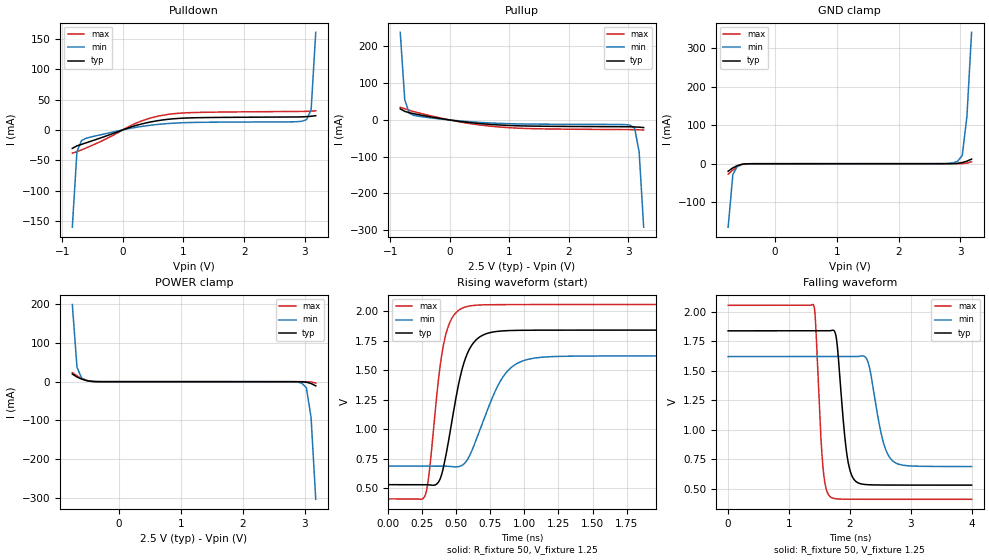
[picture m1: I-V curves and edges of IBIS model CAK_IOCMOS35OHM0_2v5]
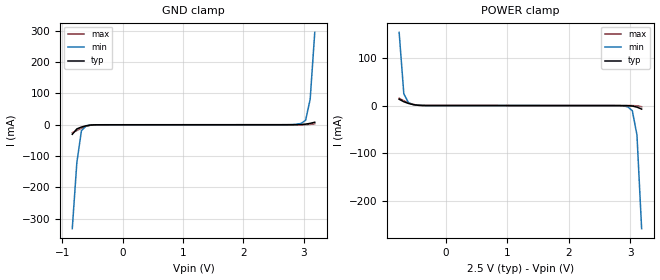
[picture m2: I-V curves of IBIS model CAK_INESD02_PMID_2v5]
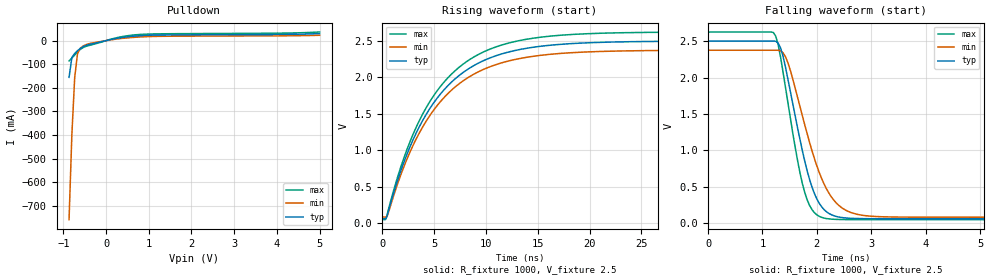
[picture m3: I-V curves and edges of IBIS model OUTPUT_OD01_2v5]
|   This file is an IBIS representation of the   |
|   Integrated Device Technology, Inc.   |
|   IDT8T49N241I   |
|   FEMTOCLOCK NG SINGLE UNIVERSAL FREQUENCY TRANSLATOR   |
[IBIS Ver]   4.1
[File name]   8t49n241i.ibs
[File Rev]   1.0
[Date]   9 Apr 2015
[Source]   Originated at Integrated Device Technology, Inc.
[Notes] This model is a based on preliminary lab data.  Typical conditions
have been correlated to lab data.  Minimum and Maximum conditions have
not been correlated to characterization data.
[Disclaimer]
IDT hereby grants the user of this IBIS model a non-exclusive,
nontransferable license to use this IBIS model under the following terms.
Before using this IBIS model, the user should read this license.
If the user does not accept these terms,  the IBIS model should be
returned to IDT within 30 days.
   The user is granted this license only to use the IBIS model and
is not granted rights to sell, load, rent, lease or license the IBIS
model in whole or in part, or in modified form to anyone other than
user. User may modify the IBIS model to suit its specific
applications but rights to derivative works and such modifications
shall belong to IDT.
   This IBIS model is provided on an "AS IS" basis and IDT makes
absolutely no warranty with respect to the information contained
herein. IDT DISCLAIMS AND CUSTOMER WAIVES ALL WARRANTIES, EXPRESS
OR IMPLIED, INCLUDING WARRANTIES OF MERCHANTABILITY OR FITNESS FOR
A PARTICULAR PURPOSE. The entire risk as to quality and performance
is with the Customer. ACCORDINGLY, IN NO EVENT SHALL THE COMPANY BE
LIABLE FOR ANY DAMAGES, WHETHER IN CONTRACT OR TORT,INCLUDING ANY
LOST PROFITS OR OTHER INCIDENTAL, CONSEQUENTIAL, EXEMPLARY, OR
PUNITIVE DAMAGES ARISING OUT OF THE USE OR APPLICATION OF THE IBIS
model provided in this package. Further, IDT reserves the right to
make changes without notice to any product herein to improve
reliability, function, or design. IDT does not convey any license
under patent rights or any other intellectual property rights,
including those of third parties.
   IDT is not obligated to provide maintenance or support
for the licensed IBIS model.
[Copyright] Copyright 2015 by Integrated Device Technology, Inc.
[Component]   IDT8T49N241NLGI
[Manufacturer] Integrated Device Technology, Inc.
[Package]
|LD QFN 40
|lead + wire   typ   min   max
R_pkg   7.1539E-02   5.8459E-02   9.5092E-02
L_pkg   1.4325E-09   1.0877E-09   2.0537E-09
C_pkg   5.9801E-14   5.5325E-14   6.5653E-14
[Pin] signal_name  model_name   R_pin   L_pin   C_pin
1   VCCA   POWER   8.5557E-02   1.8029E-09   6.3191E-14
2   VCCA   POWER   7.6183E-02   1.5542E-09   6.2015E-14
3   GPIO[0]   CAK_IOCMOS25OHM0   6.6383E-02   1.2964E-09   5.8526E-14
4   VCCO0   POWER   6.6920E-02   1.3109E-09   5.8763E-14
5   Q0   OCELL_CMOS_PECL_   6.0741E-02   1.1478E-09   5.6176E-14
6   nQ0   OCELL_CMOS_PECL_   5.8459E-02   1.0877E-09   5.5325E-14
7   GIPO[1]   CAK_IOCMOS25OHM0   6.0207E-02   1.1343E-09   5.6120E-14
8   nQ1   OCELL_CMOS_PECL_   6.3964E-02   1.2328E-09   5.7694E-14
9   Q1   OCELL_CMOS_PECL_   7.1615E-02   1.4340E-09   6.0514E-14
10  VCCO1   POWER   8.6096E-02   1.8170E-09   6.3252E-14
11  SDATA   CAK_IOCMOS35OHM0   8.6631E-02   1.8312E-09   6.3484E-14
12  SCLK   CAK_IOCMOS35OHM0   7.5512E-02   1.5366E-09   6.1638E-14
13  VCC   POWER   6.6247E-02   1.2928E-09   5.8380E-14
14  VEE   GND   6.0743E-02   1.1484E-09   5.6429E-14
15  VCC   POWER   5.9668E-02   1.1195E-09   5.5855E-14
16  CLK0   CAK_INESD02_PD   6.3966E-02   1.2326E-09   5.7537E-14
17  nCLKO   CAK_INESD02_PMID   7.3233E-02   1.4771E-09   6.1020E-14
18  CLK1   CAK_INESD02_PD   8.2496E-02   1.7204E-09   6.3925E-14
19  nCLK1   CAK_INESD02_PMID   8.5045E-02   1.7874E-09   6.4649E-14
20  S_A1   CAK_INESD01_PD   9.5092E-02   2.0537E-09   6.5653E-14
21  VCCO2   POWER   8.6362E-02   1.8241E-09   6.3205E-14
22  Q2   OCELL_CMOS_PECL_   7.0946E-02   1.4164E-09   6.0237E-14
23  nQ2   OCELL_CMOS_PECL_   6.8663E-02   1.3564E-09   5.9445E-14
24  GPIO[2]   CAK_IOCMOS25OHM0   6.5040E-02   1.2614E-09   5.8000E-14
25  nQ3   OCELL_CMOS_PECL_   6.0742E-02   1.1479E-09   5.6257E-14
26  Q3   OCELL_CMOS_PECL_   6.1547E-02   1.1691E-09   5.6462E-14
27  VCCO3   POWER   6.4102E-02   1.2369E-09   5.7655E-14
28  GPIO[3]   CAK_IOCMOS25OHM0   6.7053E-02   1.3140E-09   5.8813E-14
29  nINT   OUTPUT_OD01   7.2958E-02   1.4693E-09   6.1096E-14
30  VCCA   POWER   8.6901E-02   1.8381E-09   6.3478E-14
31  nRST   CAK_INESD01_PU   8.9987E-02   1.9196E-09   6.4336E-14
32  VCCA   POWER   8.0749E-02   1.6744E-09   6.3449E-14
33  OSCI   CAK_INESD01   6.9197E-02   1.3705E-09   5.9552E-14
34  OSCO   NC   7.0009E-02   1.3922E-09   6.0035E-14
35  nWP   CAK_INESD01_PU   6.1145E-02   1.1585E-09   5.6415E-14
36  VCCCS   POWER   5.9937E-02   1.1266E-09   5.5909E-14
37  CAP   NC   5.9804E-02   1.1237E-09   5.5979E-14
38  CAP_REF   NC   6.5441E-02   1.2716E-09   5.8175E-14
39  VCCA   POWER   7.3496E-02   1.4835E-09   6.1056E-14
40  S_A0   CAK_INESD01_PD   8.2738E-02   1.7286E-09   6.2354E-14
41  EPAD   GND
[Diff Pin]  inv_pin  vdiff tdelay_typ tdelay_min  tdelay_max
16   17   0.15   NA   NA   NA
18   19   0.15   NA   NA   NA
5   6   NA   0   0   0
9   8   NA   0   0   0
22   23   NA   0   0   0
26   25   NA   0   0   0
[Model Selector] CAK_IOCMOS25OHM0
CAK_IOCMOS25OHM0_2v5  Buffer selection for 2v5
CAK_IOCMOS25OHM0_3v3  Buffer selection for 3v3
[Model Selector] OCELL_CMOS_PECL_
OCELL_LVPECL_2v5  2.5V LVPECL Driver
OCELL_LVPECL_3v3  3.3V LVPECL Driver
OCELL_LVDS_2v5   2.5V LVDS Driver
OCELL_LVDS_3v3   3.3V LVDS Driver
OCELL_LVCMOS_1v8  1.8V LVCMOS Driver
OCELL_LVCMOS_2v5  2.5V LVCMOS Driver
OCELL_LVCMOS_3v3  3.3V LVCMOS Driver
OCELL_HCSL_2v5   2.5V HCSL Driver
OCELL_HCSL_3v3   3.3V HCSL Driver
[Model Selector] CAK_IOCMOS35OHM0
CAK_IOCMOS35OHM0_2v5  Buffer selection for 2v5
CAK_IOCMOS35OHM0_3v3  Buffer selection for 3v3
[Model Selector] CAK_INESD02_PD
CAK_INESD02_PD_2v5  Buffer selection for 2v5
CAK_INESD02_PD_3v3  Buffer selection for 3v3
[Model Selector] CAK_INESD02_PMID
CAK_INESD02_PMID_2v5  Buffer selection for 2v5
CAK_INESD02_PMID_3v3  Buffer selection for 3v3
[Model Selector] CAK_INESD01_PD
CAK_INESD01_PD_2v5  Buffer selection for 2v5
CAK_INESD01_PD_3v3  Buffer selection for 3v3
[Model Selector] OUTPUT_OD01
OUTPUT_OD01_2v5  Buffer selection for 2v5
OUTPUT_OD01_3v3  Buffer selection for 3v3
[Model Selector] CAK_INESD01_PU
CAK_INESD01_PU_2v5  Buffer selection for 2v5
CAK_INESD01_PU_3v3  Buffer selection for 3v3
[Model Selector] CAK_INESD01
CAK_INESD01_2v5  Buffer selection for 2v5
CAK_INESD01_3v3  Buffer selection for 3v3
| Models and submodels in the file (25): CAK_IOCMOS25OHM0_2v5 (Input), CAK_IOCMOS35OHM0_2v5 (I/O), CAK_INESD02_PD_2v5 (Input), CAK_INESD02_PMID_2v5 (Input), CAK_INESD01_PD_2v5 (Input), OUTPUT_OD01_2v5 (Open_drain), CAK_INESD01_PU_2v5 (Input), CAK_INESD01_2v5 (Input), CAK_IOCMOS25OHM0_3v3 (Input), OCELL_LVPECL_2v5 (Output_ECL), OCELL_LVPECL_3v3 (Output_ECL), OCELL_LVDS_2v5 (Output), OCELL_LVDS_3v3 (Output), OCELL_LVCMOS_1v8 (Output), OCELL_LVCMOS_2v5 (Output), OCELL_LVCMOS_3v3 (Output), OCELL_HCSL_2v5 (Open_source), OCELL_HCSL_3v3 (Open_source), CAK_IOCMOS35OHM0_3v3 (Output), CAK_INESD02_PD_3v3 (Input), CAK_INESD02_PMID_3v3 (Input), CAK_INESD01_PD_3v3 (Input), OUTPUT_OD01_3v3 (Open_drain), CAK_INESD01_PU_3v3 (Input), CAK_INESD01_3v3 (Input)
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| 3.18182e+00   -1.19855e-02   -3.78182e-01   -3.86041e-03
| 3.25758e+00   -2.18155e-02   -9.33967e-01   -1.12351e-02
| 3.33333e+00   -5.03193e-02   -1.56445e+00   -2.21741e-02
| 3.40909e+00   -2.87346e-01   -2.19530e+00   -3.46613e-02
| 3.48485e+00   -9.49059e-01   -2.82642e+00   -4.62600e-02
| 3.56061e+00   -1.79228e+00   -3.45775e+00   -9.04319e-02
| 3.63636e+00   -2.63582e+00   -4.08929e+00   -5.29971e-01
| 3.71212e+00   -3.47965e+00   -4.72100e+00   -1.58901e+00
| 3.78788e+00   -4.32375e+00   -5.35288e+00   -2.66834e+00
| 3.86364e+00   -5.16810e+00   -5.98493e+00   -3.74797e+00
| 3.93939e+00   -6.01268e+00   -6.61714e+00   -4.82785e+00
| 4.01515e+00   -6.85746e+00   -7.24950e+00   -5.90795e+00
| 4.09091e+00   -7.70243e+00   -7.88200e+00   -6.98824e+00
| 4.16667e+00   -8.54757e+00   -8.51465e+00   -8.06870e+00
| 4.24242e+00   -9.39286e+00   -9.14742e+00   -9.14928e+00
| 4.31818e+00   -1.02383e+01   -9.78033e+00   -1.02300e+01
| 4.39394e+00   -1.10838e+01   -1.04133e+01   -1.13108e+01
| 4.46970e+00   -1.19295e+01   -1.10465e+01   -1.23917e+01
| 4.54545e+00   -1.27752e+01   -1.16797e+01   -1.34727e+01
| 4.62121e+00   -1.36211e+01   -1.23131e+01   -1.45537e+01
| 4.69697e+00   -1.44670e+01   -1.29465e+01   -1.56349e+01
| 4.77273e+00   -1.53129e+01   -1.35800e+01   -1.67160e+01
| 4.84848e+00   -1.61590e+01   -1.42136e+01   -1.77972e+01
| 4.92424e+00   -1.70051e+01   -1.48473e+01   -1.88785e+01
| 5.00000e+00   -1.78512e+01   -1.54810e+01   -1.99597e+01
[Model] CAK_IOCMOS35OHM0_2v5
Model_type   I/O
Polarity   Non-Inverting
|   typ   min   max
C_comp   2pF   1.5pF   2.5pF
|Input
Vinl = 0.7V
Vinh = 1.7V
|Output
Vmeas = 1.25V
Rref = 50
Cref = 0
Vref = 1.25V
|   typ   min   max
[Voltage range]   2.5V   2.375V   2.625V
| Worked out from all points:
|   slope of the pulldown table from 0 to 0.375 V, typ, clamps not added: 33.2 ohm
|   slope of the pullup table from 0 to 0.375 V, typ, clamps not added: 48.8 ohm
|   GND clamp passes 1 mA (typ) near -0.50 V on its own axis
|   POWER clamp passes 1 mA (typ) near -0.46 V on its own axis
|   rising waveform, R_fixture 50, V_fixture 1.25: 20-80 % time 134ps typ, 204ps min, 96.8ps max; typ from 0.531 V to 1.84 V
|   falling waveform, R_fixture 50, V_fixture 1.25: 20-80 % time 134ps typ, 204ps min, 95ps max; typ from 1.84 V to 0.531 V
[GND_clamp]
|Voltage   I (typ)   I (min)   I (max)
|Note, modeling breaks down at 250mA and above.  This is well beyond the functional   |
|operating range of the device.  Should this scenario occur, catastrophic failure and   |
|possible damage to the device and/or board is of higher concern than the I-V curve   |
|behavior.  The IBIS checker will flag currents in excess of 10A with warnings.  Lines   |
|with currents in excess of 0.35 A have been commented out.  The points still remain|
|available to the user if the user desires to use them.   |
|-2.42424e+00   -5.99088e+00   -4.88415e+00   -7.24880e+00
|-2.34848e+00   -5.70272e+00   -4.66840e+00   -6.88094e+00
|-2.27273e+00   -5.41462e+00   -4.45272e+00   -6.51310e+00
|-2.19697e+00   -5.12656e+00   -4.23712e+00   -6.14529e+00
|-2.12121e+00   -4.83856e+00   -4.02161e+00   -5.77750e+00
|-2.04545e+00   -4.55064e+00   -3.80620e+00   -5.40975e+00
|-1.96970e+00   -4.26278e+00   -3.59088e+00   -5.04205e+00
|-1.89394e+00   -3.97502e+00   -3.37567e+00   -4.67441e+00
|-1.81818e+00   -3.68735e+00   -3.16057e+00   -4.30683e+00
|-1.74242e+00   -3.39979e+00   -2.94558e+00   -3.93934e+00
|-1.66667e+00   -3.11235e+00   -2.73072e+00   -3.57193e+00
|-1.59091e+00   -2.82505e+00   -2.51599e+00   -3.20462e+00
|-1.51515e+00   -2.53790e+00   -2.30139e+00   -2.83743e+00
|-1.43939e+00   -2.25092e+00   -2.08694e+00   -2.47036e+00
|-1.36364e+00   -1.96413e+00   -1.87263e+00   -2.10344e+00
|-1.28788e+00   -1.67754e+00   -1.65847e+00   -1.73670e+00
|-1.21212e+00   -1.39118e+00   -1.44447e+00   -1.37017e+00
|-1.13636e+00   -1.10506e+00   -1.23064e+00   -1.00389e+00
|-1.06061e+00   -8.19198e-01   -1.01701e+00   -6.37879e-01
|-9.84848e-01   -5.33627e-01   -8.03591e-01   -2.72184e-01
|-9.09091e-01   -2.48371e-01   -5.90465e-01   -5.58283e-02
|-8.33333e-01   -4.53732e-02   -3.77762e-01   -3.79192e-02
-757.6mV  -19.7mA    -165.1mA   -27.4mA
-681.8mV  -10.83mA   -28.37mA   -16.29mA
-606.1mV  -4.786mA   -6.047mA   -7.399mA
-530.3mV  -1.407mA   -1.506mA   -2.105mA
-378.8mV  -80.75uA   -97.08uA   -91.06uA
2.727V    4.903uA    107uA      2.354uA
2.879V    114.3uA    2.196mA    6.393uA
2.955V    801.8uA    6.121mA    22.36uA
3.03V     2.877mA    21.15mA    238.2uA
3.106V    6.558mA    121.9mA    1.646mA
3.182V    11.89mA    341.6mA    5.038mA
| 3.25758e+00   1.96472e-02   5.60110e-01   1.04123e-02
| 3.33333e+00   4.87507e-02   7.78570e-01   1.76749e-02
| 3.40909e+00   2.77107e-01   9.97201e-01   2.56783e-02
| 3.48485e+00   5.68788e-01   1.21604e+00   3.28468e-02
| 3.56061e+00   8.60732e-01   1.43508e+00   7.83400e-02
| 3.63636e+00   1.15296e+00   1.65434e+00   4.20975e-01
| 3.71212e+00   1.44548e+00   1.87382e+00   7.94432e-01
| 3.78788e+00   1.73828e+00   2.09351e+00   1.16825e+00
| 3.86364e+00   2.03137e+00   2.31341e+00   1.54243e+00
| 3.93939e+00   2.32473e+00   2.53352e+00   1.91695e+00
| 4.01515e+00   2.61836e+00   2.75385e+00   2.29181e+00
| 4.09091e+00   2.91225e+00   2.97438e+00   2.66701e+00
| 4.16667e+00   3.20641e+00   3.19513e+00   3.04252e+00
| 4.24242e+00   3.50082e+00   3.41608e+00   3.41834e+00
| 4.31818e+00   3.79548e+00   3.63725e+00   3.79446e+00
| 4.39394e+00   4.09039e+00   3.85863e+00   4.17087e+00
| 4.46970e+00   4.38554e+00   4.08023e+00   4.54756e+00
| 4.54545e+00   4.68094e+00   4.30204e+00   4.92452e+00
| 4.62121e+00   4.97658e+00   4.52407e+00   5.30175e+00
| 4.69697e+00   5.27245e+00   4.74633e+00   5.67924e+00
| 4.77273e+00   5.56857e+00   4.96881e+00   6.05699e+00
| 4.84848e+00   5.86492e+00   5.19152e+00   6.43499e+00
| 4.92424e+00   6.16151e+00   5.41446e+00   6.81323e+00
| 5.00000e+00   6.45834e+00   5.63765e+00   7.19172e+00
[Power_clamp]
|Voltage   I (typ)   I (min)   I (max)
|Note, modeling breaks down at 250mA and above.  This is well beyond the functional   |
|operating range of the device.  Should this scenario occur, catastrophic failure and   |
|possible damage to the device and/or board is of higher concern than the I-V curve   |
|behavior.  The IBIS checker will flag currents in excess of 10A with warnings.  Lines   |
|with currents in excess of 0.35 A have been commented out.  The points still remain|
|available to the user if the user desires to use them.   |
|-2.42424e+00   6.16151e+00   5.04673e+00   7.43787e+00
|-2.34848e+00   5.86492e+00   4.82417e+00   7.05922e+00
|-2.27273e+00   5.56857e+00   4.60184e+00   6.68082e+00
|-2.19697e+00   5.27245e+00   4.37973e+00   6.30266e+00
|-2.12121e+00   4.97658e+00   4.15784e+00   5.92475e+00
|-2.04545e+00   4.68094e+00   3.93617e+00   5.54709e+00
|-1.96970e+00   4.38554e+00   3.71471e+00   5.16969e+00
|-1.89394e+00   4.09039e+00   3.49347e+00   4.79255e+00
|-1.81818e+00   3.79548e+00   3.27244e+00   4.41568e+00
|-1.74242e+00   3.50082e+00   3.05162e+00   4.03909e+00
|-1.66667e+00   3.20641e+00   2.83101e+00   3.66278e+00
|-1.59091e+00   2.91225e+00   2.61061e+00   3.28677e+00
|-1.51515e+00   2.61836e+00   2.39042e+00   2.91105e+00
|-1.43939e+00   2.32473e+00   2.17045e+00   2.53565e+00
|-1.36364e+00   2.03137e+00   1.95069e+00   2.16057e+00
|-1.28788e+00   1.73828e+00   1.73114e+00   1.78583e+00
|-1.21212e+00   1.44548e+00   1.51180e+00   1.41142e+00
|-1.13636e+00   1.15296e+00   1.29268e+00   1.03737e+00
|-1.06061e+00   8.60732e-01   1.07377e+00   6.63681e-01
|-9.84848e-01   5.68788e-01   8.55069e-01   2.90350e-01
|-9.09091e-01   2.77107e-01   6.36557e-01   4.68087e-02
|-8.33333e-01   4.87507e-02   4.18123e-01   3.00765e-02
-757.6mV  19.65mA    199mA      23mA
-681.8mV  11.89mA    37.01mA    14.94mA
-606.1mV  6.558mA    8.981mA    8.308mA
-530.3mV  2.877mA    3.169mA    3.622mA
-303mV    14.46uA    30.61uA    12.18uA
2.727V    -54.42uA   -72.56uA   -62.76uA
2.879V    -80.75uA   -908.8uA   -66.34uA
2.955V    -281.2uA   -3.717mA   -70.88uA
3.03V     -1.407mA   -15.93mA   -127.8uA
3.106V    -4.786mA   -92.25mA   -684.1uA
3.182V    -10.83mA   -303.4mA   -3.499mA
| 3.25758e+00   -1.96989e-02   -5.15962e-01   -1.01554e-02
| 3.33333e+00   -4.53732e-02   -7.28958e-01   -2.00234e-02
| 3.40909e+00   -2.48371e-01   -9.42283e-01   -3.12866e-02
| 3.48485e+00   -5.33627e-01   -1.15585e+00   -4.17513e-02
| 3.56061e+00   -8.19198e-01   -1.36961e+00   -8.15325e-02
| 3.63636e+00   -1.10506e+00   -1.58355e+00   -4.00139e-01
| 3.71212e+00   -1.39118e+00   -1.79765e+00   -7.65947e-01
| 3.78788e+00   -1.67754e+00   -2.01191e+00   -1.13206e+00
| 3.86364e+00   -1.96413e+00   -2.22632e+00   -1.49843e+00
| 3.93939e+00   -2.25092e+00   -2.44086e+00   -1.86504e+00
| 4.01515e+00   -2.53790e+00   -2.65555e+00   -2.23184e+00
| 4.09091e+00   -2.82505e+00   -2.87037e+00   -2.59881e+00
| 4.16667e+00   -3.11235e+00   -3.08531e+00   -2.96593e+00
| 4.24242e+00   -3.39979e+00   -3.30037e+00   -3.33317e+00
| 4.31818e+00   -3.68735e+00   -3.51555e+00   -3.70052e+00
| 4.39394e+00   -3.97502e+00   -3.73083e+00   -4.06795e+00
| 4.46970e+00   -4.26278e+00   -3.94621e+00   -4.43548e+00
| 4.54545e+00   -4.55064e+00   -4.16168e+00   -4.80307e+00
| 4.62121e+00   -4.83856e+00   -4.37725e+00   -5.17074e+00
| 4.69697e+00   -5.12656e+00   -4.59290e+00   -5.53846e+00
| 4.77273e+00   -5.41462e+00   -4.80863e+00   -5.90622e+00
| 4.84848e+00   -5.70272e+00   -5.02443e+00   -6.27402e+00
| 4.92424e+00   -5.99088e+00   -5.24031e+00   -6.64184e+00
| 5.00000e+00   -6.27908e+00   -5.45625e+00   -7.00969e+00
[Pulldown]
|Voltage   I (typ)   I (min)   I (max)
|Note, modeling breaks down at 250mA and above.  This is well beyond the functional   |
|operating range of the device.  Should this scenario occur, catastrophic failure and   |
|possible damage to the device and/or board is of higher concern than the I-V curve   |
|behavior.  The IBIS checker will flag currents in excess of 10A with warnings.  Lines   |
|with currents in excess of 0.35 A have been commented out.  The points still remain|
|available to the user if the user desires to use them.   |
|-2.424240e+00   -5.620920e+00   -4.561270e+00   -6.831600e+00
|-2.348480e+00   -5.341380e+00   -4.351820e+00   -6.474360e+00
|-2.272730e+00   -5.061780e+00   -4.142370e+00   -6.117000e+00
|-2.196970e+00   -4.782250e+00   -3.932930e+00   -5.759610e+00
|-2.121210e+00   -4.502700e+00   -3.723470e+00   -5.402300e+00
|-2.045450e+00   -4.223130e+00   -3.514010e+00   -5.044950e+00
|-1.969700e+00   -3.943570e+00   -3.304540e+00   -4.687600e+00
|-1.893940e+00   -3.663980e+00   -3.095070e+00   -4.330220e+00
|-1.818180e+00   -3.384390e+00   -2.885580e+00   -3.972840e+00
|-1.742420e+00   -3.104780e+00   -2.676080e+00   -3.615430e+00
|-1.666670e+00   -2.825150e+00   -2.466570e+00   -3.258010e+00
|-1.590910e+00   -2.545490e+00   -2.257030e+00   -2.900560e+00
|-1.515150e+00   -2.265810e+00   -2.047480e+00   -2.543070e+00
|-1.439390e+00   -1.986090e+00   -1.837900e+00   -2.185550e+00
|-1.363640e+00   -1.706320e+00   -1.628300e+00   -1.827980e+00
|-1.287880e+00   -1.426520e+00   -1.418670e+00   -1.470360e+00
|-1.212120e+00   -1.146650e+00   -1.209020e+00   -1.112660e+00
|-1.136360e+00   -8.667200e-01   -9.993300e-01   -7.548700e-01
|-1.060610e+00   -5.867220e-01   -7.896000e-01   -3.969910e-01
|-9.848480e-01   -3.066460e-01   -5.798390e-01   -7.806800e-02
|-9.090910e-01   -6.551900e-02   -3.700490e-01   -4.152980e-02
-833.3mV  -30.4mA    -160.2mA   -38.37mA
-757.6mV  -26.34mA   -35.84mA   -35.89mA
-681.8mV  -23.84mA   -17.61mA   -32.95mA
-606.1mV  -21.34mA   -13.8mA    -29.8mA
227.3mV   7.551mA    4.361mA    11.42mA
454.5mV   12.99mA    7.63mA     19.37mA
681.8mV   16.67mA    9.951mA    24.52mA
1.212V    20.01mA    12.36mA    28.66mA
2.803V    21.22mA    13.27mA    30.3mA
3.03V     21.8mA     16.76mA    30.5mA
3.106V    22.45mA    33.64mA    30.79mA
3.182V    23.38mA    160.7mA    31.41mA
|3.257580e+00   2.470960e-02   3.762400e-01   3.236290e-02
|3.333330e+00   2.959920e-02   5.918100e-01   3.363400e-02
|3.409090e+00   1.001510e-01   8.074090e-01   3.503170e-02
|3.484850e+00   3.838970e-01   1.023030e+00   3.629400e-02
|3.560610e+00   6.718180e-01   1.238710e+00   4.394800e-02
|3.636360e+00   9.597900e-01   1.454410e+00   2.364620e-01
|3.712120e+00   1.247810e+00   1.670150e+00   6.046980e-01
|3.787880e+00   1.535890e+00   1.885920e+00   9.730100e-01
|3.863640e+00   1.824010e+00   2.101740e+00   1.341380e+00
|3.939390e+00   2.112190e+00   2.317600e+00   1.709840e+00
|4.015150e+00   2.400420e+00   2.533480e+00   2.078370e+00
|4.090910e+00   2.688710e+00   2.749420e+00   2.446960e+00
|4.166670e+00   2.977050e+00   2.965390e+00   2.815630e+00
|4.242420e+00   3.265440e+00   3.181400e+00   3.184380e+00
|4.318180e+00   3.553900e+00   3.397450e+00   3.553210e+00
|4.393940e+00   3.842420e+00   3.613550e+00   3.922130e+00
|4.469700e+00   4.131000e+00   3.829690e+00   4.291130e+00
|4.545450e+00   4.419630e+00   4.045870e+00   4.660220e+00
|4.621210e+00   4.708340e+00   4.262110e+00   5.029450e+00
|4.696970e+00   4.997150e+00   4.478390e+00   5.398660e+00
|4.772730e+00   5.285930e+00   4.694720e+00   5.768110e+00
|4.848480e+00   5.574880e+00   4.911080e+00   6.137610e+00
|4.924240e+00   5.863890e+00   5.127540e+00   6.507170e+00
|5.000000e+00   6.153060e+00   5.344050e+00   6.876880e+00
[Pullup]
|Voltage   I (typ)   I (min)   I (max)
|Note, modeling breaks down at 250mA and above.  This is well beyond the functional   |
|operating range of the device.  Should this scenario occur, catastrophic failure and   |
|possible damage to the device and/or board is of higher concern than the I-V curve   |
|behavior.  The IBIS checker will flag currents in excess of 10A with warnings.  Lines   |
|with currents in excess of 0.35 A have been commented out.  The points still remain|
|available to the user if the user desires to use them.   |
|-2.424240e+00   5.884990e+00   4.790360e+00   7.136830e+00
|-2.348480e+00   5.595580e+00   4.573450e+00   6.766980e+00
|-2.272730e+00   5.306130e+00   4.356560e+00   6.397080e+00
|-2.196970e+00   5.016750e+00   4.139690e+00   6.027240e+00
|-2.121210e+00   4.727390e+00   3.922850e+00   5.657350e+00
|-2.045450e+00   4.438030e+00   3.706020e+00   5.287510e+00
|-1.969700e+00   4.148680e+00   3.489220e+00   4.917710e+00
|-1.893940e+00   3.859340e+00   3.272430e+00   4.547940e+00
|-1.818180e+00   3.570020e+00   3.055660e+00   4.178140e+00
|-1.742420e+00   3.280710e+00   2.838900e+00   3.808350e+00
|-1.666670e+00   2.991410e+00   2.622170e+00   3.438570e+00
|-1.590910e+00   2.702130e+00   2.405450e+00   3.068780e+00
|-1.515150e+00   2.412850e+00   2.188750e+00   2.699010e+00
|-1.439390e+00   2.123580e+00   1.972050e+00   2.329220e+00
|-1.363640e+00   1.834310e+00   1.755360e+00   1.959430e+00
|-1.287880e+00   1.545050e+00   1.538690e+00   1.589620e+00
|-1.212120e+00   1.255770e+00   1.322030e+00   1.219810e+00
|-1.136360e+00   9.665000e-01   1.105370e+00   8.499700e-01
|-1.060610e+00   6.772080e-01   8.887100e-01   4.801090e-01
|-9.848480e-01   3.878980e-01   6.720410e-01   1.143440e-01
|-9.090910e-01   1.026590e-01   4.553330e-01   3.942970e-02
-833.3mV  30.43mA    238.5mA    34.47mA
-757.6mV  23.4mA     55.15mA    30.53mA
-681.8mV  19.94mA    18.68mA    26.41mA
-606.1mV  17.11mA    12.63mA    22.8mA
151.5mV   -3.441mA   -2.312mA   -4.819mA
833.3mV   -13.62mA   -9.198mA   -19.09mA
1.439V    -16.78mA   -11.29mA   -23.78mA
2.955V    -18.33mA   -12.6mA    -26.15mA
3.03V     -18.49mA   -13.96mA   -26.22mA
3.106V    -18.9mA    -22.45mA   -26.34mA
3.182V    -19.59mA   -87.06mA   -26.7mA
3.258V    -20.6mA    -291.6mA   -27.48mA
|3.333330e+00   -2.346490e-02   -5.006320e-01   -2.861170e-02
|3.409090e+00   -5.753200e-02   -7.096670e-01   -2.989430e-02
|3.484850e+00   -2.977200e-01   -9.187300e-01   -3.108580e-02
|3.560610e+00   -5.769620e-01   -1.127830e+00   -3.553250e-02
|3.636360e+00   -8.562400e-01   -1.336930e+00   -1.541430e-01
|3.712120e+00   -1.135550e+00   -1.546060e+00   -5.113230e-01
|3.787880e+00   -1.414880e+00   -1.755200e+00   -8.685300e-01
|3.863640e+00   -1.694240e+00   -1.964350e+00   -1.225770e+00
|3.939390e+00   -1.973620e+00   -2.173530e+00   -1.583030e+00
|4.015150e+00   -2.253020e+00   -2.382720e+00   -1.940320e+00
|4.090910e+00   -2.532440e+00   -2.591920e+00   -2.297640e+00
|4.166670e+00   -2.811880e+00   -2.801140e+00   -2.654970e+00
|4.242420e+00   -3.091330e+00   -3.010380e+00   -3.012320e+00
|4.318180e+00   -3.370810e+00   -3.219620e+00   -3.369680e+00
|4.393940e+00   -3.650300e+00   -3.428890e+00   -3.727080e+00
|4.469700e+00   -3.929810e+00   -3.638170e+00   -4.084480e+00
|4.545450e+00   -4.209330e+00   -3.847470e+00   -4.441910e+00
|4.621210e+00   -4.488880e+00   -4.056780e+00   -4.799350e+00
|4.696970e+00   -4.768440e+00   -4.266100e+00   -5.156840e+00
|4.772730e+00   -5.047980e+00   -4.475440e+00   -5.514280e+00
|4.848480e+00   -5.327580e+00   -4.684810e+00   -5.871780e+00
|4.924240e+00   -5.607220e+00   -4.894190e+00   -6.229360e+00
|5.000000e+00   -5.886920e+00   -5.103550e+00   -6.586910e+00
[Ramp]
|   typ   min   max
dV/dt_r   0.788/0.134n   0.563/0.205n   0.989/0.096n
dV/dt_f   0.788/0.134n   0.562/0.204n   0.991/0.095n
R_load =   50
[Rising Waveform]
R_fixture = 50
V_fixture = 1.25   |Vcc_typ
V_fixture_min = 1.1875 |Vcc_min
V_fixture_max = 1.3125 |Vcc_max
C_fixture = 0.0p
| Time   typ   min   max
0s        531.3mV    688.6mV    411mV
271.1ps   531.5mV    688.6mV    438.6mV
302.2ps   529.7mV    688.7mV    637.4mV
360ps     539.7mV    689mV      1.318V
408.9ps   692.4mV    688.6mV    1.728V
560ps     1.575V     710.4mV    2.033V
657.8ps   1.769V     946.1mV    2.051V
831.1ps   1.832V     1.422V     2.055V
1.031ns   1.838V     1.593V     2.056V
4ns       1.84V      1.621V     2.056V
[Falling Waveform]
R_fixture = 50
V_fixture = 1.25   |Vcc_typ
V_fixture_min = 1.1875 |Vcc_min
V_fixture_max = 1.3125 |Vcc_max
C_fixture = 0.0p
| Time   typ   min   max
0s        1.84V      1.621V     2.056V
1.404ns   1.84V      1.621V     2.057V
1.556ns   1.84V      1.621V     697.3mV
1.68ns    1.841V     1.621V     432mV
1.778ns   1.778V     1.621V     415.1mV
1.942ns   824.5mV    1.621V     412mV
2.08ns    572.1mV    1.621V     411.6mV
2.293ns   535mV      1.581V     411.3mV
2.698ns   531.9mV    739.8mV    411.1mV
4ns       531.4mV    688.9mV    411mV
| 3.25758e+00   -1.32932e-02   -4.69388e-01   -6.85289e-03
| 3.33333e+00   -3.04767e-02   -6.80964e-01   -1.35047e-02
| 3.40909e+00   -1.97405e-01   -8.92761e-01   -2.10928e-02
| 3.48485e+00   -4.80463e-01   -1.10472e+00   -2.81524e-02
| 3.56061e+00   -7.63732e-01   -1.31681e+00   -5.47589e-02
| 3.63636e+00   -1.04719e+00   -1.52902e+00   -3.40294e-01
| 3.71212e+00   -1.33083e+00   -1.74134e+00   -7.02945e-01
| 3.78788e+00   -1.61464e+00   -1.95377e+00   -1.06580e+00
| 3.86364e+00   -1.89859e+00   -2.16629e+00   -1.42883e+00
| 3.93939e+00   -2.18269e+00   -2.37891e+00   -1.79201e+00
| 4.01515e+00   -2.46691e+00   -2.59162e+00   -2.15533e+00
| 4.09091e+00   -2.75125e+00   -2.80442e+00   -2.51876e+00
| 4.16667e+00   -3.03569e+00   -3.01730e+00   -2.88228e+00
| 4.24242e+00   -3.32022e+00   -3.23027e+00   -3.24589e+00
| 4.31818e+00   -3.60483e+00   -3.44330e+00   -3.60956e+00
| 4.39394e+00   -3.88952e+00   -3.65641e+00   -3.97330e+00
| 4.46970e+00   -4.17427e+00   -3.86959e+00   -4.33710e+00
| 4.54545e+00   -4.45909e+00   -4.08283e+00   -4.70095e+00
| 4.62121e+00   -4.74395e+00   -4.29613e+00   -5.06484e+00
| 4.69697e+00   -5.02886e+00   -4.50948e+00   -5.42878e+00
| 4.77273e+00   -5.31381e+00   -4.72289e+00   -5.79275e+00
| 4.84848e+00   -5.59879e+00   -4.93635e+00   -6.15675e+00
| 4.92424e+00   -5.88381e+00   -5.14986e+00   -6.52077e+00
| 5.00000e+00   -6.16885e+00   -5.36341e+00   -6.88480e+00
[Model] CAK_INESD02_PMID_2v5
Model_type   Input
Polarity   Non-Inverting
Vinl = 0.7V
Vinh = 1.7V
|   typ   min   max
C_comp   2pF   1.5pF   2.5pF
|   typ   min   max
[Voltage range]   2.5V   2.375V   2.625V
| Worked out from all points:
|   GND clamp passes 1 mA (typ) near -0.53 V on its own axis
|   POWER clamp passes 1 mA (typ) near -0.48 V on its own axis
[GND_clamp]
|Voltage   I (typ)   I (min)   I (max)
|Note, modeling breaks down at 250mA and above.  This is well beyond the functional   |
|operating range of the device.  Should this scenario occur, catastrophic failure and   |
|possible damage to the device and/or board is of higher concern than the I-V curve   |
|behavior.  The IBIS checker will flag currents in excess of 10A with warnings.  Lines   |
|with currents in excess of 0.35 A have been commented out.  The points still remain|
|available to the user if the user desires to use them.   |
|-2.50000e+00   -6.16895e+00   -5.01116e+00   -7.48559e+00
|-2.42424e+00   -5.88390e+00   -4.79768e+00   -7.12154e+00
|-2.34848e+00   -5.59889e+00   -4.58425e+00   -6.75750e+00
|-2.27273e+00   -5.31390e+00   -4.37088e+00   -6.39347e+00
|-2.19697e+00   -5.02895e+00   -4.15756e+00   -6.02946e+00
|-2.12121e+00   -4.74404e+00   -3.94430e+00   -5.66547e+00
|-2.04545e+00   -4.45918e+00   -3.73109e+00   -5.30151e+00
|-1.96970e+00   -4.17436e+00   -3.51796e+00   -4.93758e+00
|-1.89394e+00   -3.88961e+00   -3.30490e+00   -4.57370e+00
|-1.81818e+00   -3.60492e+00   -3.09191e+00   -4.20986e+00
|-1.74242e+00   -3.32030e+00   -2.87899e+00   -3.84609e+00
|-1.66667e+00   -3.03577e+00   -2.66616e+00   -3.48237e+00
|-1.59091e+00   -2.75133e+00   -2.45342e+00   -3.11872e+00
|-1.51515e+00   -2.46699e+00   -2.24077e+00   -2.75514e+00
|-1.43939e+00   -2.18277e+00   -2.02821e+00   -2.39164e+00
|-1.36364e+00   -1.89867e+00   -1.81575e+00   -2.02825e+00
|-1.28788e+00   -1.61471e+00   -1.60339e+00   -1.66497e+00
|-1.21212e+00   -1.33091e+00   -1.39114e+00   -1.30184e+00
|-1.13636e+00   -1.04727e+00   -1.17900e+00   -9.38864e-01
|-1.06061e+00   -7.63803e-01   -9.66990e-01   -5.76078e-01
|-9.84848e-01   -4.80532e-01   -7.55130e-01   -2.13501e-01
|-9.09091e-01   -1.97473e-01   -5.43466e-01   -3.76738e-02
-833.3mV  -30.54mA   -332.1mA   -25.65mA
-757.6mV  -13.36mA   -120.7mA   -18.55mA
-681.8mV  -7.383mA   -19.06mA   -11.06mA
-606.1mV  -3.294mA   -4.129mA   -5.066mA
-530.3mV  -997.9uA   -1.06mA    -1.479mA
-378.8mV  -81.26uA   -88.94uA   -93.18uA
2.727V    59.1uA     121uA      65.12uA
2.955V    596.4uA    4.136mA    85.43uA
3.03V     1.982mA    14.16mA    231.7uA
3.106V    4.438mA    81.6mA     1.173mA
3.182V    7.992mA    295.1mA    3.436mA
| 3.25758e+00   1.31680e-02   5.12428e-01   7.02139e-03
| 3.33333e+00   3.25724e-02   7.29725e-01   1.18654e-02
| 3.40909e+00   2.27266e-01   9.47135e-01   1.72034e-02
| 3.48485e+00   5.17409e-01   1.16468e+00   2.19847e-02
| 3.56061e+00   8.07728e-01   1.38237e+00   5.23158e-02
| 3.63636e+00   1.09824e+00   1.60020e+00   3.65997e-01
| 3.71212e+00   1.38894e+00   1.81817e+00   7.37335e-01
| 3.78788e+00   1.67983e+00   2.03629e+00   1.10891e+00
| 3.86364e+00   1.97091e+00   2.25454e+00   1.48073e+00
| 3.93939e+00   2.26217e+00   2.47294e+00   1.85278e+00
| 4.01515e+00   2.55361e+00   2.69148e+00   2.22506e+00
| 4.09091e+00   2.84523e+00   2.91016e+00   2.59755e+00
| 4.16667e+00   3.13703e+00   3.12898e+00   2.97026e+00
| 4.24242e+00   3.42899e+00   3.34794e+00   3.34317e+00
| 4.31818e+00   3.72112e+00   3.56704e+00   3.71628e+00
| 4.39394e+00   4.01342e+00   3.78629e+00   4.08959e+00
| 4.46970e+00   4.30588e+00   4.00567e+00   4.46308e+00
| 4.54545e+00   4.59850e+00   4.22520e+00   4.83676e+00
| 4.62121e+00   4.89128e+00   4.44488e+00   5.21061e+00
| 4.69697e+00   5.18421e+00   4.66471e+00   5.58464e+00
| 4.77273e+00   5.47731e+00   4.88468e+00   5.95883e+00
| 4.84848e+00   5.77057e+00   5.10481e+00   6.33320e+00
| 4.92424e+00   6.06399e+00   5.32510e+00   6.70773e+00
| 5.00000e+00   6.35756e+00   5.54554e+00   7.08242e+00
[Power_clamp]
|Voltage   I (typ)   I (min)   I (max)
|Note, modeling breaks down at 250mA and above.  This is well beyond the functional   |
|operating range of the device.  Should this scenario occur, catastrophic failure and   |
|possible damage to the device and/or board is of higher concern than the I-V curve   |
|behavior.  The IBIS checker will flag currents in excess of 10A with warnings.  Lines   |
|with currents in excess of 0.35 A have been commented out.  The points still remain|
|available to the user if the user desires to use them.   |
|-2.50000e+00   6.35756e+00   5.18189e+00   7.70102e+00
|-2.42424e+00   6.06399e+00   4.96171e+00   7.32606e+00
|-2.34848e+00   5.77057e+00   4.74168e+00   6.95126e+00
|-2.27273e+00   5.47731e+00   4.52180e+00   6.57663e+00
|-2.19697e+00   5.18421e+00   4.30207e+00   6.20215e+00
|-2.12121e+00   4.89128e+00   4.08249e+00   5.82785e+00
|-2.04545e+00   4.59850e+00   3.86306e+00   5.45371e+00
|-1.96970e+00   4.30588e+00   3.64376e+00   5.07974e+00
|-1.89394e+00   4.01342e+00   3.42461e+00   4.70595e+00
|-1.81818e+00   3.72112e+00   3.20560e+00   4.33234e+00
|-1.74242e+00   3.42899e+00   2.98673e+00   3.95891e+00
|-1.66667e+00   3.13703e+00   2.76800e+00   3.58567e+00
|-1.59091e+00   2.84523e+00   2.54941e+00   3.21263e+00
|-1.51515e+00   2.55361e+00   2.33097e+00   2.83979e+00
|-1.43939e+00   2.26217e+00   2.11266e+00   2.46715e+00
|-1.36364e+00   1.97091e+00   1.89450e+00   2.09473e+00
|-1.28788e+00   1.67983e+00   1.67647e+00   1.72254e+00
|-1.21212e+00   1.38894e+00   1.45859e+00   1.35057e+00
|-1.13636e+00   1.09824e+00   1.24086e+00   9.78833e-01
|-1.06061e+00   8.07728e-01   1.02326e+00   6.07339e-01
|-9.84848e-01   5.17409e-01   8.05803e-01   2.36085e-01
|-9.09091e-01   2.27266e-01   5.88473e-01   3.12941e-02
|-8.33333e-01   3.25724e-02   3.71194e-01   2.01370e-02
-757.6mV  13.17mA    153.4mA    15.42mA
-681.8mV  7.992mA    24.73mA    10.04mA
-606.1mV  4.438mA    6.043mA    5.618mA
-530.3mV  1.982mA    2.167mA    2.491mA
-303mV    67.49uA    68.92uA    77.83uA
2.727V    -58.92uA   -71.21uA   -65.12uA
2.955V    -222.7uA   -2.559mA   -77.6uA
3.03V     -997.9uA   -10.75mA   -119.7uA
3.106V    -3.295mA   -61.69mA   -506.7uA
3.182V    -7.383mA   -258.2mA   -2.426mA
| 3.25758e+00   -2.17677e-02   -5.28452e-01   -1.11757e-02
| 3.33333e+00   -5.02723e-02   -7.41922e-01   -2.21158e-02
| 3.40909e+00   -2.62314e-01   -9.55756e-01   -3.46040e-02
| 3.48485e+00   -5.48303e-01   -1.16986e+00   -4.62037e-02
| 3.56061e+00   -8.34641e-01   -1.38418e+00   -9.03765e-02
| 3.63636e+00   -1.12130e+00   -1.59869e+00   -4.17028e-01
| 3.71212e+00   -1.40825e+00   -1.81339e+00   -7.83888e-01
| 3.78788e+00   -1.69546e+00   -2.02826e+00   -1.15108e+00
| 3.86364e+00   -1.98293e+00   -2.24329e+00   -1.51857e+00
| 3.93939e+00   -2.27062e+00   -2.45848e+00   -1.88632e+00
| 4.01515e+00   -2.55852e+00   -2.67383e+00   -2.25428e+00
| 4.09091e+00   -2.84661e+00   -2.88932e+00   -2.62244e+00
| 4.16667e+00   -3.13486e+00   -3.10494e+00   -2.99075e+00
| 4.24242e+00   -3.42327e+00   -3.32071e+00   -3.35921e+00
| 4.31818e+00   -3.71181e+00   -3.53659e+00   -3.72777e+00
| 4.39394e+00   -4.00047e+00   -3.75260e+00   -4.09645e+00
| 4.46970e+00   -4.28924e+00   -3.96871e+00   -4.46521e+00
| 4.54545e+00   -4.57811e+00   -4.18494e+00   -4.83406e+00
| 4.62121e+00   -4.86706e+00   -4.40126e+00   -5.20297e+00
| 4.69697e+00   -5.15608e+00   -4.61767e+00   -5.57195e+00
| 4.77273e+00   -5.44517e+00   -4.83417e+00   -5.94098e+00
| 4.84848e+00   -5.73432e+00   -5.05076e+00   -6.31005e+00
| 4.92424e+00   -6.02353e+00   -5.26742e+00   -6.67914e+00
| 5.00000e+00   -6.31277e+00   -5.48416e+00   -7.04826e+00
[Model] OUTPUT_OD01_2v5
Model_type   Open_drain
Polarity   Non-Inverting
|   typ   min   max
C_comp   2pF   1.5pF   2.5pF
Vmeas = 0.729V
Rref = 1000
Cref = 0
Vref = 2.5V
|   typ   min   max
[Voltage range]   2.5V   2.375V   2.625V
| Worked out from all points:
|   slope of the pulldown table from 0 to 0.375 V, typ, clamps not added: 28.6 ohm
|   rising waveform, R_fixture 1000, V_fixture 2.5: 20-80 % time 5.89ns typ, 5.96ns min, 5.83ns max; typ from 0.058 V to 2.5 V
|   falling waveform, R_fixture 1000, V_fixture 2.5: 20-80 % time 429ps typ, 552ps min, 357ps max; typ from 2.5 V to 0.058 V
[Pulldown]
|Note, modeling breaks down at 250mA and above.  This is well beyond the functional   |
|operating range of the device.  Should this scenario occur, catastrophic failure and   |
|possible damage to the device and/or board is of higher concern than the I-V curve   |
|behavior.  The IBIS checker will flag currents in excess of 10A with warnings.  Lines   |
|with currents in excess of 0.35 A have been commented out.  The points still remain|
|available to the user if the user desires to use them.   |
|Voltage   I (typ)   I (min)   I (max)
|-2.50000e+00   -1.22461e+01   -9.96179e+00   -1.48391e+01
|-2.20000e+00   -9.99080e+00   -8.26740e+00   -1.19637e+01
|-1.90000e+00   -7.73621e+00   -6.57432e+00   -9.08860e+00
|-1.60000e+00   -5.48288e+00   -4.88287e+00   -6.21429e+00
|-1.30000e+00   -3.23142e+00   -3.19335e+00   -3.34148e+00
|-1.00000e+00   -9.82636e-01   -1.50618e+00   -4.75877e-01
|-9.99000e-01   -9.75146e-01   -1.50057e+00   -4.67694e-01
|-9.32920e-01   -4.81499e-01   -1.12938e+00   -1.28883e-01
-866.8mV  -155.7mA   -758.5mA   -85.96mA
-800.8mV  -71.35mA   -397.8mA   -73.72mA
-734.7mV  -54.25mA   -156.2mA   -60.9mA
-668.6mV  -42.8mA    -55.01mA   -48.03mA
-602.5mV  -33.2mA    -32.01mA   -37.18mA
-536.4mV  -25.63mA   -22.78mA   -29.3mA
-338.2mV  -14.09mA   -10.49mA   -17.88mA
256.5mV   9.624mA    6.792mA    12.56mA
785.2mV   20.77mA    15.36mA    26mA
4.155V    26.3mA     20.4mA     31.86mA
5V        29.84mA    22.63mA    36.62mA
[Ramp]
|   typ   min   max
dV/dt_r   1.465/5.892n   1.377/5.96n   1.548/5.829n
dV/dt_f   1.465/0.429n   1.377/0.551n   1.548/0.357n
R_load =   50.0000
[Rising Waveform]
R_fixture = 1000
V_fixture = 2.5
V_fixture_min = 2.375
V_fixture_max = 2.625
C_fixture = 0.0p
| Time   typ   min   max
0s        58.29mV    79.84mV    46.07mV
311.1ps   57.79mV    78.84mV    47.72mV
488.9ps   110.1mV    101.3mV    127.2mV
2.356ns   935.8mV    869.4mV    1.001V
4.489ns   1.551V     1.456V     1.645V
6.933ns   1.969V     1.858V     2.08V
9.911ns   2.24V      2.119V     2.36V
13.33ns   2.386V     2.262V     2.51V
18.09ns   2.464V     2.339V     2.589V
40ns      2.5V       2.375V     2.625V
[Falling Waveform]
R_fixture = 1000
V_fixture = 2.5
V_fixture_min = 2.375
V_fixture_max = 2.625
C_fixture = 0.0p
| Time   typ   min   max
0s        2.5V       2.375V     2.625V
1.2ns     2.501V     2.375V     2.618V
1.289ns   2.473V     2.375V     2.45V
1.422ns   2.148V     2.287V     1.867V
1.778ns   850.6mV    1.348V     419.3mV
2ns       331.2mV    786.1mV    112.7mV
2.267ns   114.3mV    359.8mV    53.56mV
2.667ns   63.52mV    134.7mV    46.87mV
3.467ns   58.72mV    82.36mV    46.27mV
40ns      58.3mV     79.85mV    46.07mV
